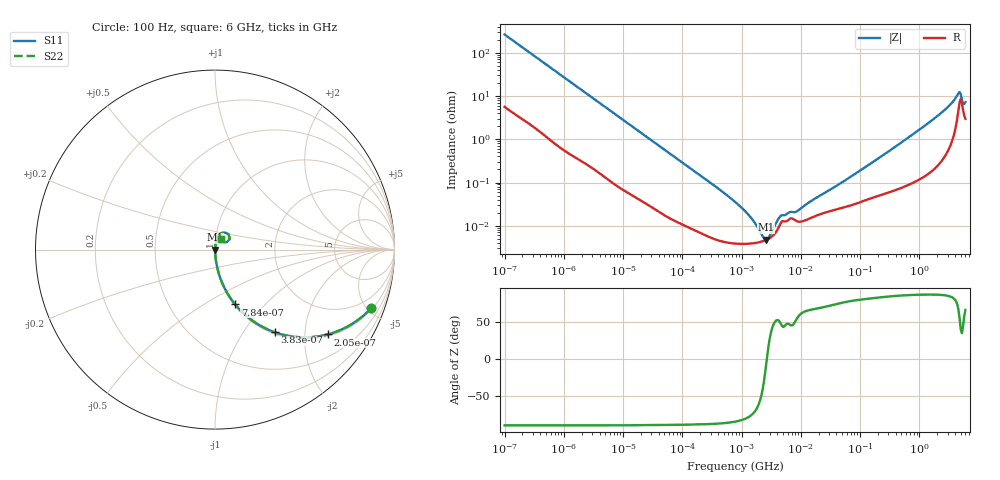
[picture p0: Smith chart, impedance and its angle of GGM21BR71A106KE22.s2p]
!Murata Part Number: GGM21BR71A106KE22
!These Parameters are Measured in Series Mode Connection
!Data Generated on Jun 19, 2026
!  o--ll--o
!Port1  Port2
!  o------o
!Operation Temp=25[degC], DC Bias Voltage=0[V]
!Freq. Start=100[Hz] Stop=6[GHz] 401[Steps]
# Hz S RI R 50
!Freq.(Hz) S11(Real) S11(Imag) S21(Real) S21(Imag) S12(Real) S12(Imag) S22(Real) S22(Imag)
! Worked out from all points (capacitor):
!   401 points, 100 Hz to 6 GHz, reference 50 ohm
!   read as one part in series: C = 5.99 uF near 109 Hz
!   lowest |Z| = 4.73 mohm at 2.595 MHz (marker M1)
!   series resonance near 2.665 MHz, so ESL is about 600 pH
!   S11 on the Smith chart (normalised r, x): 100 Hz: 1.11, -5.29; 205 Hz: 1.06, -2.61; 383 Hz: 1.03, -1.41; 784 Hz: 1.01, -0.69; 6 GHz: 1.06, +0.13
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100  0.8697 -0.3262  0.1303 0.3262  0.1303 0.3262  0.8697 -0.3262
205  0.6271 -0.4728  0.3729 0.4728  0.3729 0.4728  0.6271 -0.4728
383  0.3345 -0.461  0.6655 0.461  0.6655 0.461  0.3345 -0.461
784  0.1123 -0.3057  0.8877 0.3057  0.8877 0.3057  0.1123 -0.3057
2008  0.0213 -0.1336  0.9787 0.1336  0.9787 0.1336  0.0213 -0.1336
6433  0.00289 -0.0434  0.9971 0.0434  0.9971 0.0434  0.00289 -0.0434
40335  0.000259 -0.00713  0.9997 0.00713  0.9997 0.00713  0.000259 -0.00713
774597  3.88e-05 -0.000356  1 0.000356  1 0.000356  3.88e-05 -0.000356
1212075  3.82e-05 -0.000198  1 0.000198  1 0.000198  3.82e-05 -0.000198
1813585  4.06e-05 -9.02e-05  1 9.02e-05  1 9.02e-05  4.06e-05 -9.02e-05
2594782  4.69e-05 -6.2e-06  1 6.2e-06  1 6.2e-06  4.69e-05 -6.2e-06
3394479  5.95e-05 5.87e-05  0.9999 -5.87e-05  0.9999 -5.87e-05  5.95e-05 5.87e-05
4643984  0.000119 0.000125  0.9999 -0.000125  0.9999 -0.000125  0.000119 0.000125
8692127  0.000126 0.000178  0.9999 -0.000178  0.9999 -0.000178  0.000126 0.000178
1.555665e7  0.000157 0.000355  0.9998 -0.000355  0.9998 -0.000355  0.000157 0.000355
3.124326e8  0.000624 0.00535  0.9994 -0.00535  0.9994 -0.00535  0.000624 0.00535
2.142435e9  0.00395 0.0364  0.996 -0.0364  0.996 -0.0364  0.00395 0.0364
3.205649e9  0.00964 0.0585  0.9904 -0.0585  0.9904 -0.0585  0.00964 0.0585
4.385646e9  0.0393 0.0931  0.9607 -0.0931  0.9607 -0.0931  0.0393 0.0931
4.796499e9  0.0754 0.0858  0.9246 -0.0858  0.9246 -0.0858  0.0754 0.0858
5.486059e9  0.047 0.0421  0.953 -0.0421  0.953 -0.0421  0.047 0.0421
6e9  0.0328 0.0616  0.9672 -0.0616  0.9672 -0.0616  0.0328 0.0616
